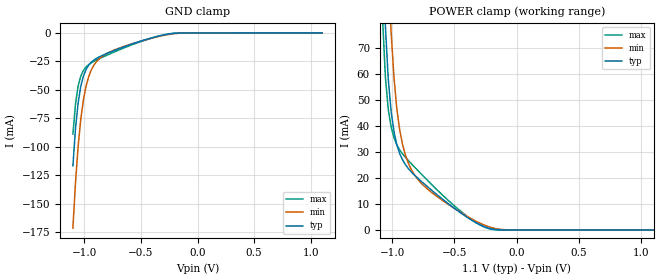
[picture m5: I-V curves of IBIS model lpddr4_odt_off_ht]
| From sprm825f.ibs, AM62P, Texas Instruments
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|   Model lpddr4_odt_off_ht
[Model] lpddr4_odt_off_ht
Model_type Input
Polarity   Non-Inverting
Enable   Active-High
Vinl =  0.113V
Vinh =  0.253V
C_comp   2.926pF   2.918pF   2.927pF
[Model Spec]
Vinh   0.253V   0.247V   0.265V
Vinl   0.113V   0.107V   0.125V
[Temperature Range]   25.000   0.125k   -40.000
[Voltage Range]   1.100V   1.060V   1.170V
[C Comp Corner]
C_comp   2.927pF   2.926pF   2.918pF
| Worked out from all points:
|   GND clamp passes 1 mA (typ) near -0.26 V on its own axis
|   POWER clamp passes 1 mA (typ) near -0.24 V on its own axis
[GND_clamp]
|Voltage   I(typ)   I(min)   I(max)
-1.1V     -116.8mA   -171.6mA   -88.94mA
-1.077V   -83.94mA   -131.3mA   -62.39mA
-1.054V   -61.59mA   -99.85mA   -46.82mA
-1.031V   -47.19mA   -76.32mA   -38.12mA
-1.008V   -38.15mA   -59.31mA   -33.14mA
-985mV    -32.43mA   -47.29mA   -30.06mA
-940mV    -26.01mA   -32.94mA   -26.4mA
-894mV    -22.49mA   -25.52mA   -23.93mA
-848mV    -20.1mA    -21.14mA   -21.77mA
-619mV    -11.19mA   -10.92mA   -11.99mA
-229mV    -598.7uA   -1.002mA   -573.1uA
1.1V      0A         0A         0A
[POWER_clamp]
|Voltage   I(typ)   I(min)   I(max)
-1.1V     158.5mA    248.7mA    122.8mA
-1.077V   110.5mA    184.5mA    81.82mA
-1.054V   78.44mA    136mA      58.83mA
-1.031V   58.13mA    100.8mA    46.38mA
-1.008V   45.62mA    75.96mA    39.55mA
-985mV    37.81mA    58.73mA    35.43mA
-963mV    32.84mA    46.93mA    32.79mA
-940mV    29.44mA    38.73mA    30.81mA
-871mV    23.66mA    25.79mA    26.72mA
-642mV    13.63mA    12.95mA    15.53mA
-206mV    448.9uA    953.6uA    285.7uA
1.1V      0A         0A         0A
